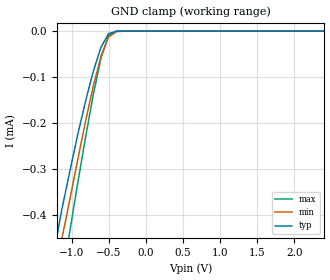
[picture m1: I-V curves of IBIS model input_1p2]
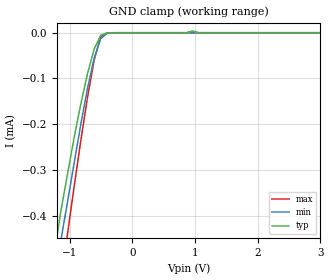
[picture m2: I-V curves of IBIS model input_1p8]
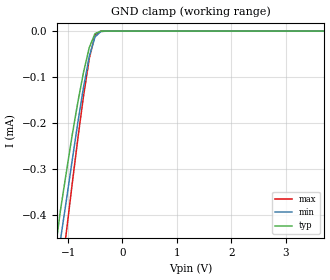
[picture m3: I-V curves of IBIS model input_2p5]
| Texas Instruments Incorporated
| TXU0104 4-Bit Fixed Direction Voltage-Level Translator
| with 3-State outputs and Schmitt-trigger Inputs
[IBIS Ver]   4.1
[File name]   txu0104.ibs
[File Rev]   1.0
[Date]   03/29/2021
[Source]
| Texas Instruments Incorporated.
| Analog-eLab Design Center, HPA
| 12500 TI Blvd
| Dallas, TX -75243
[Notes]   Revision History:
| Rev 1.0: 03/29/2021
| - Initial version of the model
| - Model generated from simulations in SPECTRE
| - C_comp although listed in numerical order of value are
|   obtained from varying PVT conditions. For PVT conditions for
|   each specific value refer the buffer description under
|   respective [Model]. IBIS model user is responsible for using
|   appropriate C_comp to simulate for Signal Integrity.
| - Warnings regarding combined Non-monotonicity of various models have been
|   reviewed and are considered minor and can be ignored.
| - Model names with a trailing _2p5 contain the model for 2.5V operation.
[Disclaimer]
| This model is designed as an aid for customers of Texas Instruments.
| TI and its licensors and suppliers make no warranties, either expressed
| or implied, with respect to this  model, including the warranties of
| merchantability or fitness for a particular purpose. The model is
| provided solely on an "as is" basis. The entire risk as to its quality
| and performance is with the customer.
| This model is subject to change without notice. Texas Instruments
| Incorporated is not responsible for updating this model.
[Copyright]
 (C) Copyright 2021 Texas Instruments Incorporated.All rights reserved.
|  Component TXU0104PW 14-Pin TSSOP - PW package
|  Part # TXU0104PWR
[Component]   TXU0104PW
[Manufacturer]   TI
[Package]   |14 TSSOP - PW package
|   typ   min   max
R_pkg   3.900e-02   3.000e-02   4.600e-02
L_pkg   2.685e-09   2.367e-09   3.177e-09
C_pkg   3.200e-13   2.520e-13   4.340e-13
[Pin]   signal_name   model_name   R_pin   L_pin   C_pin
1   VCCA   power   3.700e-02   3.153e-09   4.340e-13
2   A1   input   4.200e-02   2.741e-09   2.900e-13
3   A2   input   4.200e-02   2.741e-09   2.900e-13
4   A3   input   4.200e-02   2.741e-09   2.900e-13
5   A4   input   4.600e-02   2.600e-09   2.620e-13
6   NC   NC   4.300e-02   2.414e-09   2.660e-13
7   GND   gnd   3.700e-02   2.670e-09   3.460e-13
8   OE   input   3.100e-02   2.738e-09   3.390e-13
9   NC   NC   4.300e-02   2.414e-09   2.660e-13
10   B4Y   output   4.400e-02   2.425e-09   2.660e-13
11   B3Y   output   4.400e-02   2.425e-09   2.660e-13
12   B2Y   output   4.600e-02   2.532e-09   2.570e-13
13   B1Y   output   4.200e-02   2.648e-09   2.820e-13
14   VCCB   power   3.600e-02   2.653e-09   3.440e-13
|  Component TXU0104BQA 14-Pin WQFN - BQA package
|  Part # TXU0104BQAR
[Component]   TXU0104BQA
[Manufacturer]   TI
[Package]   |14 WQFN - BQA package
|   typ   min   max
R_pkg   3.700e-02   2.500e-02   5.300e-02
L_pkg   8.060e-10   5.310e-10   1.139e-09
C_pkg   1.880e-13   5.700e-14   3.100e-13
[Pin]   signal_name   model_name   R_pin   L_pin   C_pin
1   VCCA   power   3.700e-02   3.153e-09   4.340e-13
2   A1   input   4.200e-02   2.741e-09   2.900e-13
3   A2   input   4.200e-02   2.741e-09   2.900e-13
4   A3   input   4.200e-02   2.741e-09   2.900e-13
5   A4   input   4.600e-02   2.600e-09   2.620e-13
6   NC   NC   4.300e-02   2.414e-09   2.660e-13
7   GND   gnd   3.700e-02   2.670e-09   3.460e-13
8   OE   input   3.100e-02   2.738e-09   3.390e-13
9   NC   NC   4.300e-02   2.414e-09   2.660e-13
10   B4Y   output   4.400e-02   2.425e-09   2.660e-13
11   B3Y   output   4.400e-02   2.425e-09   2.660e-13
12   B2Y   output   4.600e-02   2.532e-09   2.570e-13
13   B1Y   output   4.200e-02   2.648e-09   2.820e-13
14   VCCB   power   3.600e-02   2.653e-09   3.440e-13
|  Component TXU0104RUT 12-Pin UQFN - RUT package
|  Part # TXU0104RUTR
[Component]   TXU0104RUT
[Manufacturer]   TI
[Package]   |12 UQFN - RUT package
|   typ   min   max
R_pkg   3.700e-02   2.500e-02   5.300e-02
L_pkg   8.060e-10   5.310e-10   1.139e-09
C_pkg   1.880e-13   5.700e-14   3.100e-13
[Pin]   signal_name   model_name   R_pin   L_pin   C_pin
1   VCCA   power   3.700e-02   3.153e-09   4.340e-13
2   A1   input   4.200e-02   2.741e-09   2.900e-13
3   A2   input   4.200e-02   2.741e-09   2.900e-13
4   A3   input   4.200e-02   2.741e-09   2.900e-13
5   A4   input   4.600e-02   2.600e-09   2.620e-13
6   GND   gnd   3.700e-02   2.670e-09   3.460e-13
7   OE   input   3.100e-02   2.738e-09   3.390e-13
8   B4Y   output   4.400e-02   2.425e-09   2.660e-13
9   B3Y   output   4.400e-02   2.425e-09   2.660e-13
10   B2Y   output   4.600e-02   2.532e-09   2.570e-13
11   B1Y   output   4.200e-02   2.648e-09   2.820e-13
12   VCCB   power   3.600e-02   2.653e-09   3.440e-13
|  Component TXU0104DTR 12-Pin X2SON - DTR package
|  Part # TXU0104DTRR
[Component]   TXU0104DTR
[Manufacturer]   TI
[Package]   |12 X2SON - DTR package
|   typ   min   max
R_pkg   3.700e-02   2.500e-02   5.300e-02
L_pkg   8.060e-10   5.310e-10   1.139e-09
C_pkg   1.880e-13   5.700e-14   3.100e-13
[Pin]   signal_name   model_name   R_pin   L_pin   C_pin
1   VCCA   power   3.700e-02   3.153e-09   4.340e-13
2   A1   input   4.200e-02   2.741e-09   2.900e-13
3   A2   input   4.200e-02   2.741e-09   2.900e-13
4   A3   input   4.200e-02   2.741e-09   2.900e-13
5   A4   input   4.600e-02   2.600e-09   2.620e-13
6   GND   gnd   3.700e-02   2.670e-09   3.460e-13
7   OE   input   3.100e-02   2.738e-09   3.390e-13
8   B4Y   output   4.400e-02   2.425e-09   2.660e-13
9   B3Y   output   4.400e-02   2.425e-09   2.660e-13
10   B2Y   output   4.600e-02   2.532e-09   2.570e-13
11   B1Y   output   4.200e-02   2.648e-09   2.820e-13
12   VCCB   power   3.600e-02   2.653e-09   3.440e-13
|   Model Selectors
[Model Selector] input
input_1p2   1.2V   digital input
input_1p8   1.8V   digital input
input_2p5   2.5V   digital input
input_3p3   3.3V   digital input
input_5p0   5.0V   digital input
[Model Selector] output
output_1p2   1.2V   digital output
output_1p8   1.8V   digital output
output_2p5   2.5V   digital output
output_3p3   3.3V   digital output
output_5p0   5.0V   digital output
| Models and submodels in the file (10): input_1p2 (Input), input_1p8 (Input), input_2p5 (Input), input_3p3 (Input), input_5p0 (Input), output_1p2 (Output), output_1p8 (Output), output_2p5 (Output), output_3p3 (Output), output_5p0 (Output)
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|   input_1p2 Model
[Model]   input_1p2
Model_type   Input
Vinl = 0.2
Vinh = 0.9
|   typ   min   max
C_comp   0.119pF   0.105pF   0.126pF
[Voltage Range]   1.2   1.08   1.32
|Junction Temperature
[Temperature Range]   25   125   -40
[GND Clamp Reference]   0   0   0
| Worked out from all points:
|   GND clamp passes 1 mA (typ) near -1.81 V on its own axis
[GND Clamp]
|   Voltage   I(typ)   I(min)   I(max)
-2.5V     -1.66mA    -1.64mA    -2.09mA
-1.24V    -478uA     -541uA     -650uA
-1.14V    -389uA     -453uA     -542uA
-1.03V    -305uA     -366uA     -435uA
-925mV    -226uA     -281uA     -332uA
-820mV    -154uA     -198uA     -233uA
-715mV    -88.7uA    -121uA     -140uA
-610mV    -35.6uA    -54.9uA    -59.7uA
-505mV    -5.5uA     -12.7uA    -8.49uA
-400mV    -210nA     -1.13uA    -141nA
8V        3.62nA     3.43nA     4.23nA
|   input_1p8 Model
[Model]   input_1p8
Model_type   Input
Vinl = 0.7
Vinh = 1.1
|   typ   min   max
C_comp   3.13pF   2.65pF   3.82pF
| Where Nom  PVT is Nominal Process, 2.25V, 27C
|   Fast PVT is Strong Process,  2.50V, -55C
|   Slow PVT is Weak Process,   2.0V, 150C
[Voltage Range]   1.8   1.62   1.98
|Junction Temperature
[Temperature Range]   25   125   -40
[GND Clamp Reference]   0   0   0
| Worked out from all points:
|   GND clamp passes 1 mA (typ) near -1.81 V on its own axis
[GND Clamp]
|   Voltage   I(typ)   I(min)   I(max)
-2.5V     -1.66mA    -1.64mA    -2.09mA
-1.24V    -478uA     -541uA     -650uA
-1.14V    -389uA     -453uA     -542uA
-1.03V    -305uA     -366uA     -435uA
-820mV    -154uA     -198uA     -233uA
-715mV    -88.7uA    -121uA     -140uA
-610mV    -35.6uA    -54.9uA    -59.7uA
-505mV    -5.5uA     -12.7uA    -8.49uA
-400mV    -210nA     -1.13uA    -141nA
965mV     3.74uA     3.02nA     4.93nA
1.07V     3.25nA     2.95nA     3.92nA
8V        3.62nA     3.43nA     4.23nA
|   input_2p5 Model
[Model]   input_2p5
Model_type   Input
Vinl = 1.0
Vinh = 1.4
|   typ   min   max
C_comp   3.03pF   2.54pF   3.83pF
| Where Nom  PVT is Nominal Process, 2.25V, 27C
|   Fast PVT is Strong Process,  2.50V, -55C
|   Slow PVT is Weak Process,   2.0V, 150C
[Voltage Range]   2.5   2.25   2.75
|Junction Temperature
[Temperature Range]   25   125   -40
[GND Clamp Reference]   0   0   0
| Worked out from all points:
|   GND clamp passes 1 mA (typ) near -1.81 V on its own axis
[GND Clamp]
|   Voltage   I(typ)   I(min)   I(max)
-2.5V     -1.66mA    -1.64mA    -2.09mA
-1.24V    -478uA     -541uA     -650uA
-1.14V    -389uA     -453uA     -542uA
-1.03V    -305uA     -366uA     -435uA
-925mV    -226uA     -281uA     -332uA
-820mV    -154uA     -198uA     -233uA
-715mV    -88.7uA    -121uA     -140uA
-610mV    -35.6uA    -54.9uA    -59.7uA
-505mV    -5.5uA     -12.7uA    -8.49uA
-400mV    -210nA     -1.14uA    -141nA
8V        3.62nA     3.43nA     4.23nA
